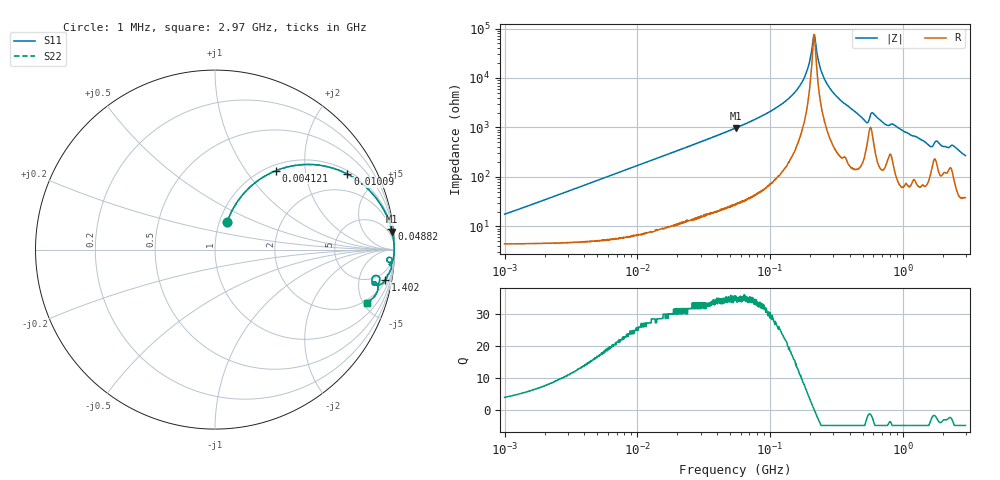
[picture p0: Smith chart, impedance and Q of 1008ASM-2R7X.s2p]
!s-Parameter Generated by FASTRON Sdn. Bhd.
!FASTRON P/N : 1008ASM-2R7X
!Keysight Technologies: E4991B_MY54100416_A.01.15
!Date: Tue Nov 21 10:09:47 2023
!Version  :Rev00  Wed Nov 22 15:09:32 2023
!Data & Calibration Information:
!Freq  S11  S21  S12  S22
!PortZ  Port1:50+j0  Port2:50+j0
!When reading reference impedance value at option line is always used.
! Remarks : This data is being provided solely for informational purposes.
# Hz S dB R 50
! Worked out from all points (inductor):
!   1599 points, 1 MHz to 2.97 GHz, reference 50 ohm
!   read as one part in series: L = 2.72 uH near 1.036 MHz
!   highest Q = 35.1 at 55.6 MHz (marker M1), where L = 2.81 uH
!   self-resonance near 214.7 MHz
!   S11 on the Smith chart (normalised r, x): 1 MHz: 1.09, +0.34; 4.121 MHz: 1.10, +1.40; 10.09 MHz: 1.13, +3.42; 48.82 MHz: 1, +17; 1.402 GHz: 2, -11; 2.97 GHz: 1.76, -5.35
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1000000  -15.50 66.1  -0.49 -9.3  -0.49 -9.3  -15.50 66.1
3804036  -5.56 54.0  -1.82 -31.7  -1.82 -31.7  -5.56 54.0
4121125  -5.08 52.2  -2.02 -33.8  -2.02 -33.8  -5.08 52.2
1.009296e7  -1.42 29.7  -6.10 -58.1  -6.10 -58.1  -1.42 29.7
1.439846e7  -0.78 22.0  -8.54 -66.0  -8.54 -66.0  -0.78 22.0
4.881767e7  -0.09 6.7  -18.70 -81.7  -18.70 -81.7  -0.09 6.7
5.477226e7  -0.07 5.9  -19.80 -82.5  -19.80 -82.5  -0.07 5.9
5.56007e7  -0.07 5.8  -19.90 -82.6  -19.90 -82.6  -0.07 5.8
1.018679e8  -0.02 2.6  -26.70 -85.4  -26.70 -85.4  -0.02 2.6
1.497525e8  -0.01 1.2  -33.50 -85.3  -33.50 -85.3  -0.01 1.2
1.847772e8  -0.01 0.5  -41.10 -81.2  -41.10 -81.2  -0.01 0.5
2.073156e8  -0.01 0.1  -52.00 -58.5  -52.00 -58.5  -0.01 0.1
2.168657e8  -0.01 -0.0  -57.10 19.1  -57.10 19.1  -0.01 -0.0
2.349428e8  -0.01 -0.3  -45.60 74.7  -45.60 74.7  -0.01 -0.3
2.507343e8  -0.01 -0.5  -41.00 80.3  -41.00 80.3  -0.01 -0.5
3.285236e8  -0.02 -1.5  -31.80 84.4  -31.80 84.4  -0.02 -1.5
5.284703e8  -0.20 -4.2  -22.40 70.7  -22.40 70.7  -0.20 -4.2
5.929311e8  -0.16 -2.7  -26.10 67.1  -26.10 67.1  -0.16 -2.7
7.846996e8  -0.21 -5.0  -21.00 72.0  -21.00 72.0  -0.21 -5.0
1.402151e9  -0.33 -10.0  -15.20 72.9  -15.20 72.9  -0.33 -10.0
2.383164e9  -0.70 -11.8  -13.50 62.9  -13.50 62.9  -0.70 -11.8
2.970126e9  -0.94 -19.2  -9.58 62.7  -9.58 62.7  -0.94 -19.2
